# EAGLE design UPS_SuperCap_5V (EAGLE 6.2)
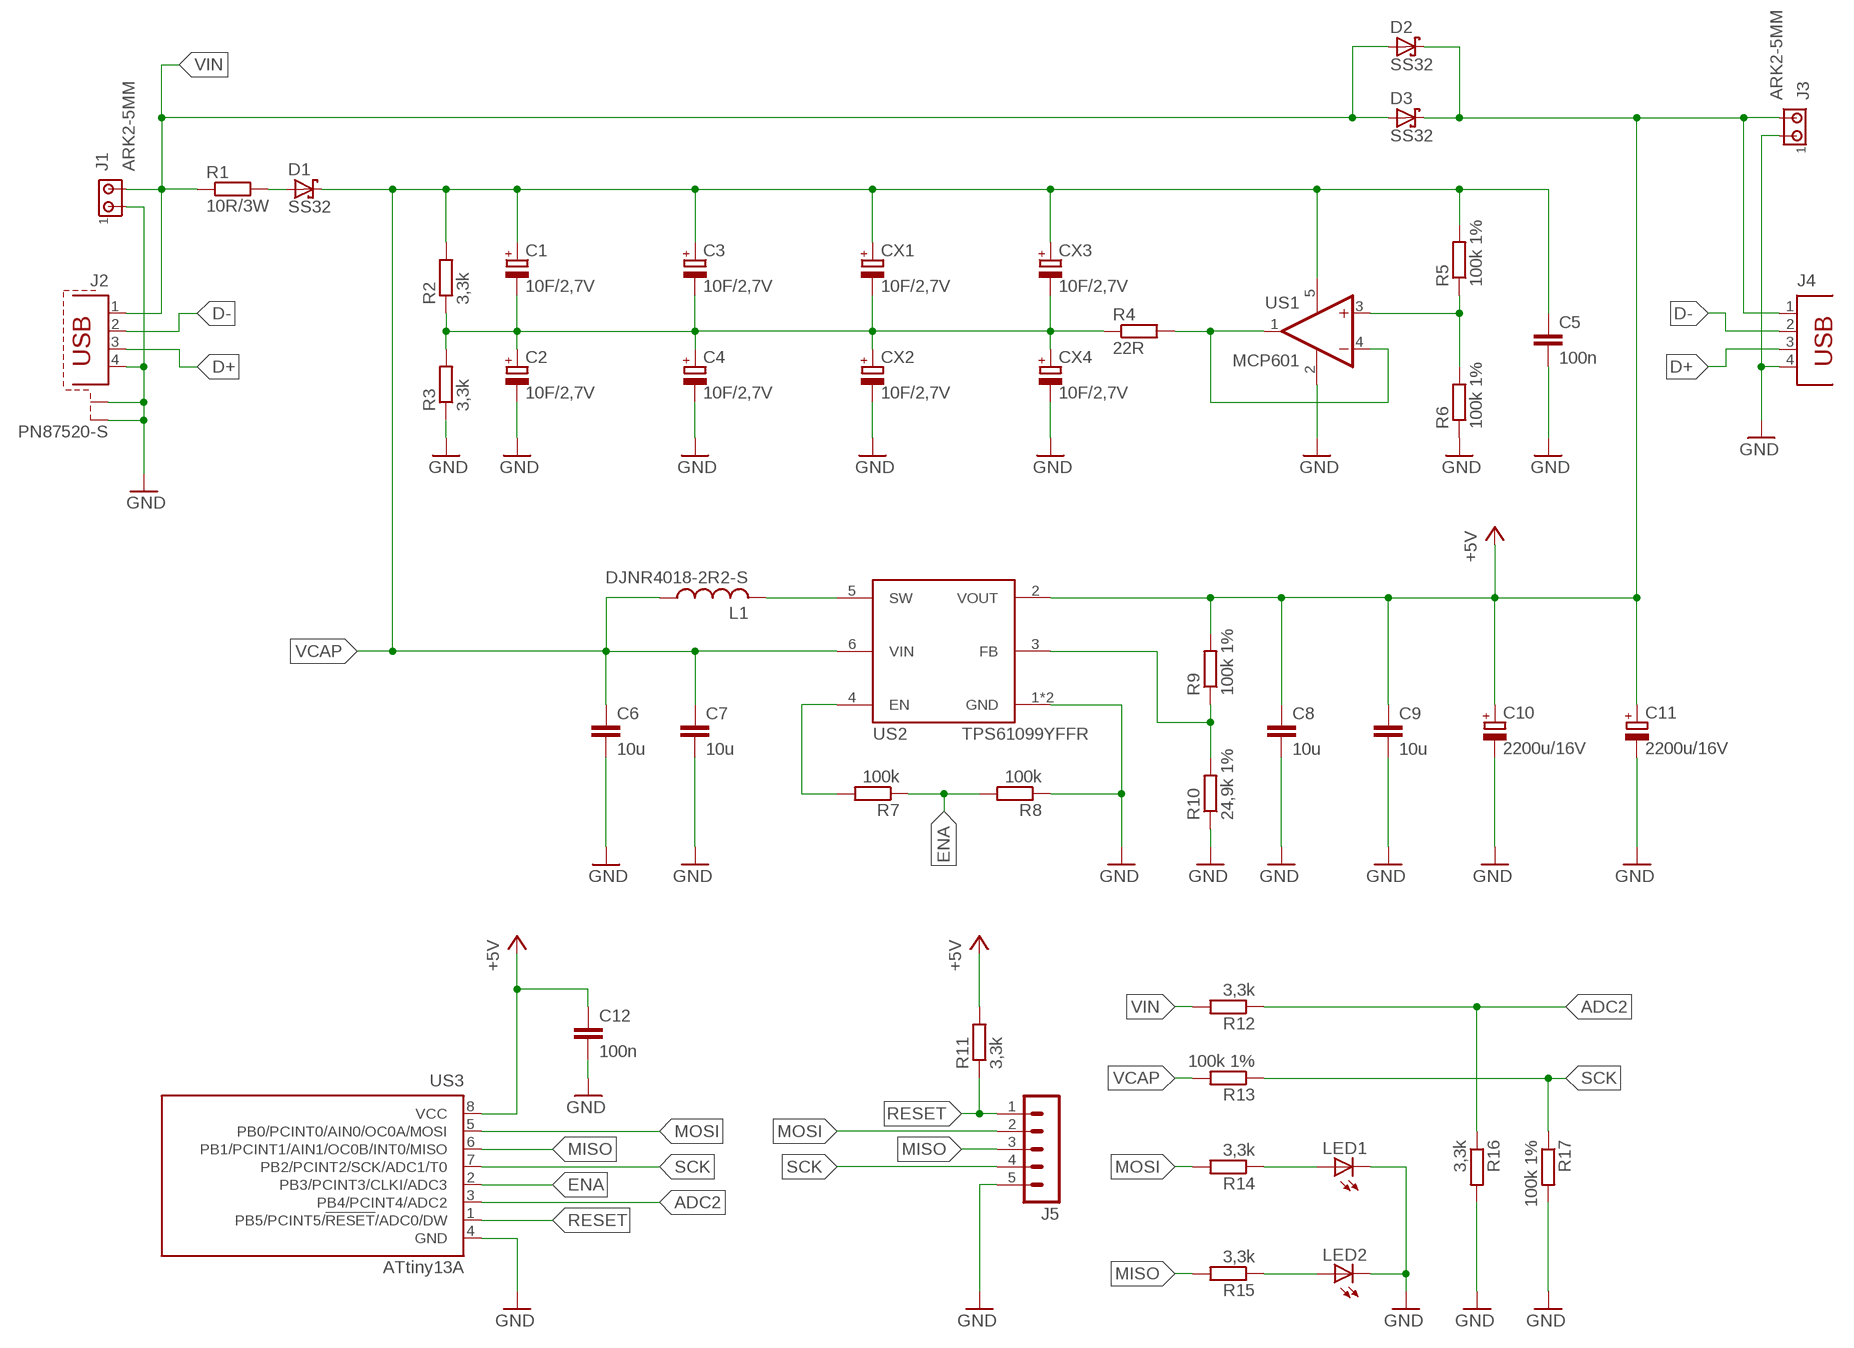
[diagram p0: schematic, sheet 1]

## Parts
C1  10F/2,7V  CPOL-EUE5-13  [E5-13]
C2  10F/2,7V  CPOL-EUE5-13  [E5-13]
C3  10F/2,7V  CPOL-EUE5-13  [E5-13]
C4  10F/2,7V  CPOL-EUE5-13  [E5-13]
C5  100n  C-EUC0805  [C0805]
C6  10u  C-EUC0805  [C0805]
C7  10u  C-EUC0805  [C0805]
C8  10u  C-EUC0805  [C0805]
C9  10u  C-EUC0805  [C0805]
C10  2200u/16V  CPOL-EUE5-10.5  [E5-10,5]
C11  2200u/16V  CPOL-EUE5-10.5  [E5-10,5]
C12  100n  C-EUC0805  [C0805]
CX1  10F/2,7V  CPOL-EUE5-13  [E5-13]
CX2  10F/2,7V  CPOL-EUE5-13  [E5-13]
CX3  10F/2,7V  CPOL-EUE5-13  [E5-13]
CX4  10F/2,7V  CPOL-EUE5-13  [E5-13]
D1  SS32  SCHOTTKY-DIODESMC  [SMC]
D2  SS32  SCHOTTKY-DIODESMC  [SMC]
D3  SS32  SCHOTTKY-DIODESMC  [SMC]
J1  ARK2-5MM  [2PIN-5MM]
J2  PN87520-S  [PN87520-S]
J3  ARK2-5MM  [2PIN-5MM]
J4  PN87520  [PN87520]
J5  MA05-1  [MA05-1]
L1  DJNR4018-2R2-S  L-USWE-TPC  [POWER-CHOKE_WE-TPC]
LED1  LEDCHIPLED_0805  [CHIPLED_0805]
LED2  LEDCHIPLED_0805  [CHIPLED_0805]
R1  10R/3W  R-EU_0817/7V  [P0817V]
R2  3,3k  R-EU_R0805  [R0805]
R3  3,3k  R-EU_R0805  [R0805]
R4  22R  R-EU_R1206  [R1206]
R5  100k 1%  R-EU_R0805  [R0805]
R6  100k 1%  R-EU_R0805  [R0805]
R7  100k  R-EU_R0805  [R0805]
R8  100k  R-EU_R0805  [R0805]
R9  100k 1%  R-EU_R0805  [R0805]
R10  24,9k 1%  R-EU_R0805  [R0805]
R11  3,3k  R-EU_R0805  [R0805]
R12  3,3k  R-EU_R0805  [R0805]
R13  100k 1%  R-EU_R0805  [R0805]
R14  3,3k  R-EU_R0805  [R0805]
R15  3,3k  R-EU_R0805  [R0805]
R16  3,3k  R-EU_R0805  [R0805]
R17  100k 1%  R-EU_R0805  [R0805]
US1  MCP601  MCP601OT  [SOT23-5]
US2  TPS61099YFFR  TPS61099  [DSBGA6]
US3  ATtiny13A  TINY13V-10SSU  [8S1]

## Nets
+5V: C8.1 C9.1 C10.+ C11.+ C12.1 D2.C D3.C J3.P$2 J4.1 R9.2 R11.2 US2.2(VOUT) US3.8(VCC)
ADC2: R12.1 R16.1 US3.3(PB4/PCINT4/ADC2)
D+: J2.3 J4.3
D-: J2.2 J4.2
ENA: R7.1 R8.2 US3.2(PB3/PCINT3/CLKI/ADC3)
GND: C2.- C4.- C5.2 C6.2 C7.2 C8.2 C9.2 C10.- C11.- C12.2 CX2.- CX4.- J1.P$1 J2.4 J2.S1 J2.S2 J3.P$1 J4.4 J5.5 LED1.C LED2.C R3.1 R6.1 R8.1 R10.1 R16.2 R17.2 US1.2(V-) US2.1(GND) US2.7(GND) US3.4(GND)
MISO: J5.3 R15.2 US3.6(PB1/PCINT1/AIN1/OC0B/INT0/MISO)
MOSI: J5.2 R14.2 US3.5(PB0/PCINT0/AIN0/OC0A/MOSI)
N$1: LED1.A R14.1
N$2: C1.- C2.+ C3.- C4.+ CX1.- CX2.+ CX3.- CX4.+ R2.1 R3.2 R4.1
N$3: L1.2 US2.5(SW)
N$4: R4.2 US1.1(OUT) US1.4(-IN)
N$5: R5.1 R6.2 US1.3(+IN)
N$6: LED2.A R15.1
N$7: R9.1 R10.2 US2.3(FB)
N$8: D1.A R1.2
N$9: R7.2 US2.4(EN)
RESET: J5.1 R11.1 US3.1(PB5/PCINT5/!RESET!/ADC0/DW)
SCK: J5.4 R13.1 R17.1 US3.7(PB2/PCINT2/SCK/ADC1/T0)
VCAP: C1.+ C3.+ C5.1 C6.1 C7.1 CX1.+ CX3.+ D1.C L1.1 R2.2 R5.2 R13.2 US1.5(V+) US2.6(VIN)
VIN: D2.A D3.A J1.P$2 J2.1 R1.1 R12.2

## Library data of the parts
C1-C4 C10 C11 CX1-CX4 = rcl:CPOL-EU: POLARIZED CAPACITOR, European symbol
C5-C9 C12 = resistor:C-EU: CAPACITOR, European symbol
D1-D3 = diode:SCHOTTKY-DIODE: Schottky Diode
J1 J3 = zlacza_futrzak:ARK2: ARK 2
J2 = zlacza_futrzak:PN87520-S; OC_FARNELL: unknown; OC_NEWARK: unknown
J4 = con-berg:PN87520: BERG USB connector; OC_FARNELL: unknown; OC_NEWARK: unknown
J5 = zlacza_futrzak:MA05-1: PIN HEADER; OC_FARNELL: unknown; OC_NEWARK: unknown
L1 = rcl:L-US: INDUCTOR, American symbol
LED1 LED2 = led:LED: LED
R1 = rcl:R-EU_: RESISTOR, European symbol
R2-R17 = resistor:R-EU_: RESISTOR, European symbol
US1 = linear:MCP601: Single Op Amp 2.7V to 6.0V Single Supply CMOS Source: http://ww1.microchip.com/downloads/en/DeviceDoc/21314g.pdf
US2 = scalaki_futrzak:TPS61099
US3 = atmel:TINY13: 8-bit AVR Microcontroller with 1K Bytes In-System Programmable Flash Source: http://www.atmel.com/dyn/resources/prod_documents/2535S.pdf; MPN: ATTINY13V-10SSU; OC_FARNELL: 1455135; OC_NEWARK: 58M3773

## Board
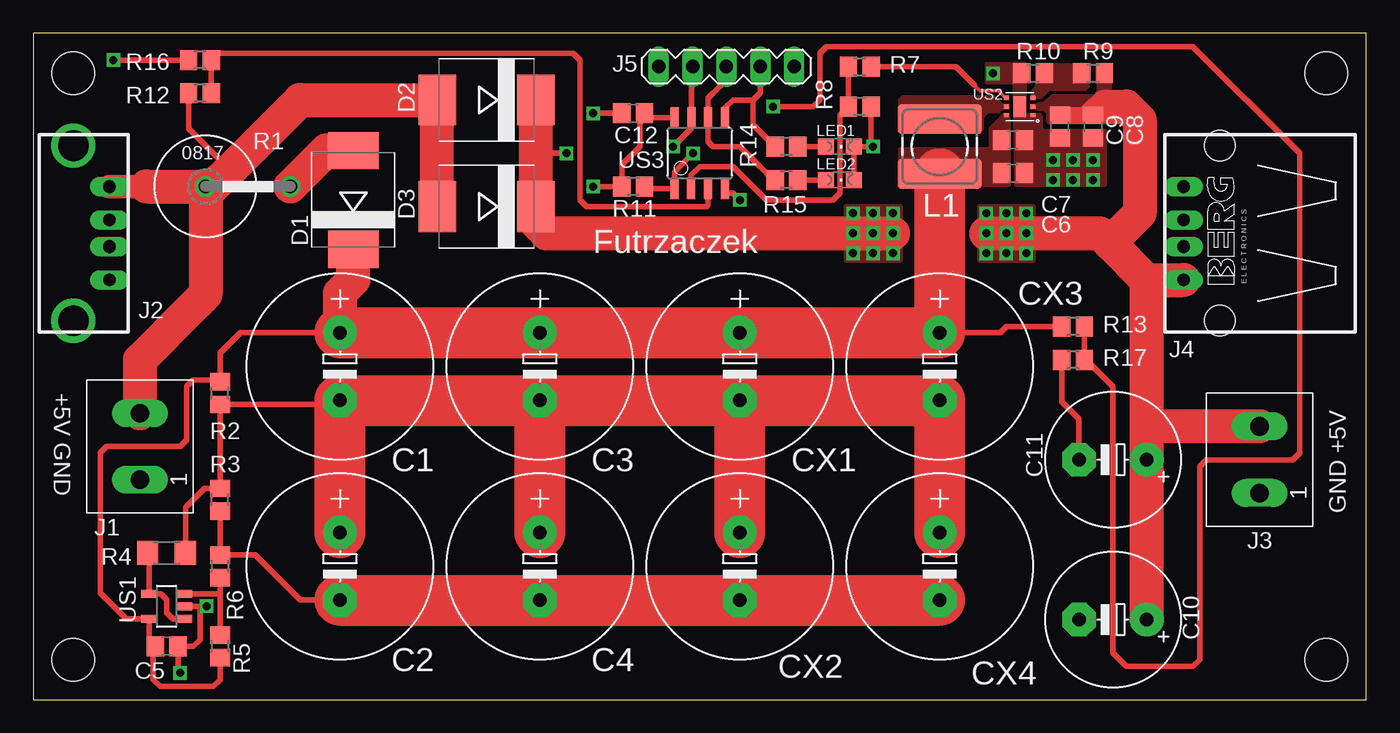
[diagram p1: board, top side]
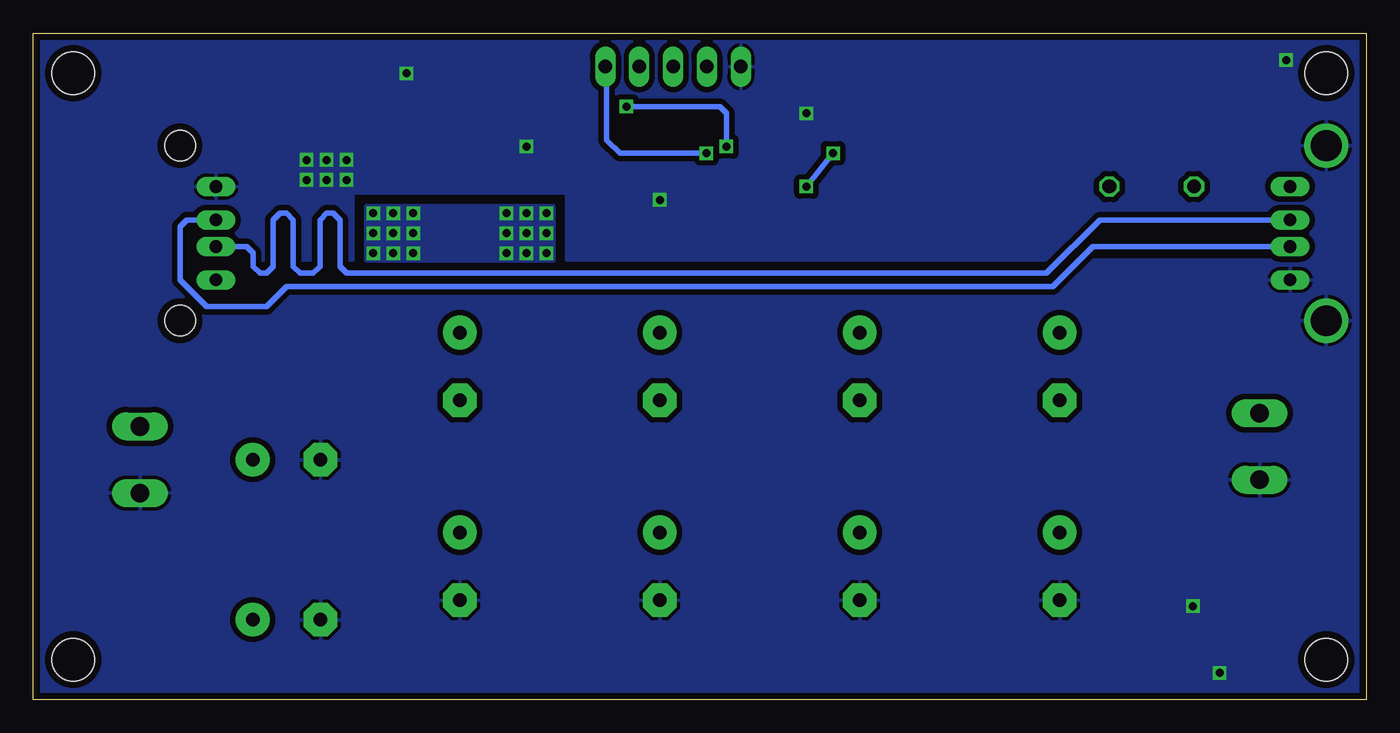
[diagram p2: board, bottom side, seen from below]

Size 100 x 50 mm. Coordinates in mm from the lower left corner, seen from the top.
Outline: 0,0 100,0 100,50 0,50 0,0
Copper layers (1*16): Top 0.035mm / dielectric 1.5mm / Bottom 0.035mm
Design rules: minimum track width 10mil, minimum drill 23mil, track to track 8mil, track to pad 8mil, pad to pad 8mil, via to via 8mil, smd to smd 8mil, copper to edge 20mil, drill to drill 8mil, minimum pad ring 10mil, minimum via ring 8mil, stop-mask expansion 4mil, vias tented up to drill 0mil, thermal gap 10mil
Holes 3.2 mm at 3,3 3,47 97,47 97,3

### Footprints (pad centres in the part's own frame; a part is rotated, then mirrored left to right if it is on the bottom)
E5-13 = drill 1.016 pad 2.54: + -2.54,0 | drill 1.016 pad 2.54 octagon: - 2.54,0
C0805 = smd 1.3 x 1.5: 1 -0.85,0; 2 0.85,0
E5-10,5 = drill 1.016 pad 2.54: + -2.54,0 | drill 1.016 pad 2.54 octagon: - 2.54,0
SMC = smd 2.8 x 3.8: A 3.7,0; C -3.7,0
2PIN-5MM = drill 1.4 long: P$1 -2.5,0; P$2 2.5,0
PN87520-S = drill 0.95 long: 1 -3.5,2.71; 2 -1,2.71; 3 1,2.71; 4 3.5,2.71 | drill 2.3 pad 2.9: S1 -6.57,0; S2 6.57,0
PN87520 = drill 0.95 long: 1 -3.5,2.71; 2 -1,2.71; 3 1,2.71; 4 3.5,2.71 | hole 2.3: -6.57,0; 6.57,0
MA05-1 = drill 1.016 long: 1 -5.08,0; 2 -2.54,0; 3 0,0; 4 2.54,0; 5 5.08,0
POWER-CHOKE_WE-TPC = smd 6.3 x 2.2: 1 0,2.05; 2 0,-2.05
CHIPLED_0805 = smd 1.2 x 1.2: A 0,-1.05; C 0,1.05
P0817V = drill 1.016 octagon: 1 -5.08,0; 2 1.27,0
R0805 = smd 1.3 x 1.5: 1 -0.85,0; 2 0.85,0
R1206 = smd 1.6 x 1.803: 1 -1.422,0; 2 1.422,0
SOT23-5 = smd 0.6 x 1.2: 1 -0.95,-1.306; 2 0,-1.306; 3 0.95,-1.306; 4 0.95,1.306; 5 -0.95,1.306
DSBGA6 = smd 0.45 x 0.3: 1 -1,0.65; 2 -1,0; 3 -1,-0.65; 4 1,-0.65; 5 1,0; 6 1,0.65 | smd 1 x 1.6: 7 0,0
8S1 = smd 0.6 x 1.6: 1 -1.905,-2.654; 2 -0.645,-2.654; 3 0.625,-2.654; 4 1.895,-2.654; 5 1.905,2.654; 6 0.635,2.654; 7 -0.635,2.654; 8 -1.905,2.654

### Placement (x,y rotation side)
C1  23,25 270 top
C2  23,10 270 top
C3  38,25 270 top
C4  38,10 270 top
C5  10,4 0 top
C6  73.5,42 0 top
C7  73.5,39.5 0 top
C8  77,43 270 top
C9  79.5,43 270 top
C10  81,6 180 top
C11  81,18 180 top
C12  45,44 180 top
CX1  53,25 270 top
CX2  53,10 270 top
CX3  68,25 270 top
CX4  68,10 270 top
D1  24,37.5 90 top
D2  34,45 180 top
D3  34,37 180 top
J1  8,19 90 top
J2  3,35 270 top
J3  92,18 90 top
J4  89,35 90 top
J5  52,47.5 180 top
L1  68,41.5 180 top
LED1  60.5,41.5 270 top
LED2  60.5,39 270 top
R1  18,38.5 0 top
R2  14,23 90 top
R3  14,15 90 top
R4  10,11 180 top
R5  14,4 270 top
R6  14,10 270 top
R7  62,47.5 0 top
R8  62,44.5 180 top
R9  79.5,47 0 top
R10  75,47 0 top
R11  45,38.5 180 top
R12  12.5,45.5 180 top
R13  78,28 180 top
R14  56.5,41.5 180 top
R15  56.5,39 180 top
R16  12.5,48 180 top
R17  78,25.5 180 top
US1  10,7 90 top
US2  74,44.5 180 top
US3  50,41 0 top

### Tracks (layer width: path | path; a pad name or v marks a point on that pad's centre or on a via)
+5V  (via drill 0.6)
  Top 0.406: v42,38.5 R11.2 44.15,40.15 45.5,41.5 45.5,43.65 C12.1 46.2,43.65 US3.8 | v40,41 37.7,41
  Top 1.27: C8.1 78.85,43.85 79.5,44.5 80.5,44.5
  Top 2.54: D2.C 37.7,41 D3.C 37.7,35.8 38.5,35 v64.5,35 | v71.5,35 80,35 80.75,34.25 | 80.75,34.25 83.5,31.5 | 83.5,31.5 J4.1 | 83.54,20.5 C11.+ C10.+ | 83.54,20.5 83.54,31.46 83.5,31.5 | J3.P$2 83.54,20.5 | 80.5,44.5 82,44.5 83,43.5 83,36.5 80.75,34.25
  Bottom 0.406: v42,38.5 v40,41
  other vias: 63,35 61.5,35 73,35 74.5,35 64.5,36.5 63,36.5 61.5,36.5 71.5,36.5 73,36.5 74.5,36.5 61.5,33.5 63,33.5 64.5,33.5 71.5,33.5 73,33.5 74.5,33.5
  pour Top (isolate 0.254, no thermals): 80.6,43.3 76.2,43.3 76.1,43.4 76.1,44 75.8,44.3 74.8,44.3 74.8,44.7 75.8,44.7 76.4,45.3 79.6,45.3 79.9,45.6 79.9,47.6 80.8,47.6 80.8,43.5
  pour Bottom (isolate 0.406, no thermals): 61,37 75,37 75,33 61,33
  pour Top (isolate 0.406, no thermals): 61,37 65,37 65,33 61,33
  pour Top (isolate 0.406, no thermals): 71,37 75,37 75,33 71,33
ADC2
  Top 0.406: R12.1 13.35,47.85 | 13.35,47.85 13.5,48.5 40.5,48.5 41,48 41,37.5 41.5,37 50.5,37 50.62,37.12 US3.3 | 13.35,47.85 R16.1
D+
  Bottom 0.406: J4.3 88.5,36 89,35.5 89,31.5 87,29.5 82.5,29.5 81,31 23.5,31 20.5,34 J2.3
D-
  Bottom 0.406: J4.2 84,34 83.5,33.5 83.5,32.5 83,32 82.5,32 82,32.5 82,36 81.5,36.5 81,36.5 80.5,36 80.5,32.5 80,32 79,32 78.5,32.5 78.5,36 78,36.5 77.5,36.5 77,36 77,32.5 76.5,32 24,32 20,36 J2.2
ENA
  Top 0.406: US3.2 49.35,39.35 50,40 52.5,40 55,37.5 60,37.5 60.5,38 60.5,43.85 R8.2 R7.1
GND  (via drill 0.6)
  Top 0.406: LED2.C LED1.C v63,41.5 62.85,41.65 R8.1 | C12.2 v42,44 | v53,37.5 52.5,38 52,38 52,38.24 US3.4 | US1.2 12.5,7 | 12.5,7 v13,7 | v11,2 10.85,2.15 C5.2 12,4 12.5,4.5 12.5,7 | C2.- 22.96,7.5 20,7.5 16.65,10.85 R6.1 R3.1 | R17.2 77.15,22.35 78.46,21.04 C11.- | R16.2 v6,48
  Top 3.81: C2.- C4.- CX2.- CX4.-
  other vias: 72,47 76.5,40.5 78,40.5 79.5,40.5 76.5,39 78,39 79.5,39
  pour Top (isolate 0.254, no thermals): 73.7,38.6 80.4,38.6 80.4,42.7 75.8,42.7 75.6,42.9 75.6,43.8 75.5,43.9 74.4,43.9 74.4,47.7 71.5,47.7 71.5,46.3 73.6,46.3
  pour Bottom (isolate 0.406): 0,33 60,33 60,38 76,38 76,33 100,33 100,50 0,50
  pour Bottom (isolate 0.406): 0,33 60,33 60,32 76,32 76,33 100,33 100,0 0,0
MISO
  Top 0.406: J5.3 52,46.5 51,45.5 50.63,45.13 US3.6 50.63,42.37 50.63,41.87 51,41.5 53,41.5 54.5,40 55.5,39 R15.2
MOSI
  Top 0.406: US3.5 51.91,44.41 52.5,45 54,45 | J5.2 54.54,45.54 54,45 | 54,45 54,43.15 R14.2
N$1
  Top 0.406: LED1.A R14.1
N$2
  Top 0.406: C1.- 22.69,22.15 R2.1 R3.2 12.85,15.85 12.5,15.5 11.42,14.42 R4.1
  Top 3.81: C2.+ C1.- C3.- | C4.+ C3.- | CX2.+ CX1.- | C3.- CX1.- | CX1.- 67.5,22.46 | 67.5,22.46 CX3.- | CX4.+ 68,21.96 67.5,22.46
N$3
  pour Top (isolate 0.254, no thermals): 71.2,43.7 71.6,44.1 73.3,44.1 73.3,44.8 72.5,44.8 72.1,45.2 65.2,45.2 65,45 65,42.7 65.1,42.6 71,42.6 71.2,42.8
N$4
  Top 0.406: R4.2 8.69,10.88 US1.4 9.55,7.95 10,7.5 10,6.5 10.45,6.05 US1.1
N$5
  Top 0.406: R5.1 14,8 | 14,8 R6.2 | US1.3 13.95,7.95 14,8
N$6
  Top 0.406: LED2.A R15.1
N$7
  pour Top (isolate 0.254, no thermals): 75.6,45.2 75,45.2 75,45.7 75.3,46 75.3,47.6 79.1,47.6 79.1,46 78.9,45.8 76.2,45.8
N$8
  Top 2.54: D1.A 21.97,41.2 R1.2
N$9
  Top 0.254: US2.4 72.95,45.15 72.4,45.7 71,45.7 70.6,46.1
  Top 0.406: 70.6,46.1 69.8,46.9 69.2,47.5 R7.2
RESET  (via drill 0.6)
  Top 0.406: R11.1 46,38.35 US3.1 48.09,39.59 v49.5,41
  Bottom 0.406: v49.5,41 56,41 57,42 57,47.42 J5.1
SCK  (via drill 0.6)
  Top 0.406: J5.4 49.37,47.41 US3.7 49.37,42.87 v48,41.5 | R13.1 78.85,25.65 | 78.85,25.65 81,23.5 81,3.5 82,2.5 87,2.5 87.5,3 87.5,17.5 88,18 94.5,18 95,18.5 95,41 87,49 59.5,49 59,48.5 59,45 58.5,44.5 v55.5,44.5 | 78.85,25.65 R17.1
  Bottom 0.406: v55.5,44.5 48.5,44.5 48,44 v48,41.5
VCAP
  Top 0.406: R13.2 73,28 72.54,27.54 CX3.+ | R5.2 14,1.5 13.5,1 9.5,1 9,1.5 9,3.85 C5.1 8.69,4.46 US1.5 6.95,6.05 5,8 5,18.5 5.5,19 11,19 11.5,19.5 11.5,23.5 12,24 13.85,24 R2.2 14,26 15.54,27.54 C1.+
  Top 2.54: C1.+ 23,30.5 24,31.5 D1.C
  Top 3.81: C1.+ C3.+ CX1.+ CX3.+ L1.1
  pour Top (isolate 0.254, no thermals): 72.8,43.9 73.2,43.9 73.2,38.6 65,38.6 65,41.3 71.6,41.3 71.8,41.5 71.8,42.9
VIN
  Top 0.406: R12.2 11.65,42.85 14.75,39.75 15,39.5
  Top 1.778: J2.1 8.5,38.5
  Top 2.54: D3.A D2.A 20,45 14.75,39.75 13.5,38.5 R1.1 | 8.5,38.5 R1.1 | J1.P$2 8,25.5 12,29.5 12.5,30 12.92,30.42 R1.1

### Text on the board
tPlace: Futrzaczek | +5V GND | GND +5V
